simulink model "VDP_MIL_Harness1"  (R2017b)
settings: Solver=FixedStepDiscrete  StartTime=0.0  StopTime=50  FixedStep=0.01  RelTol=1e-3  EnableMultiTasking=on
undefined symbols (not defined in the file): sigbuilder_block

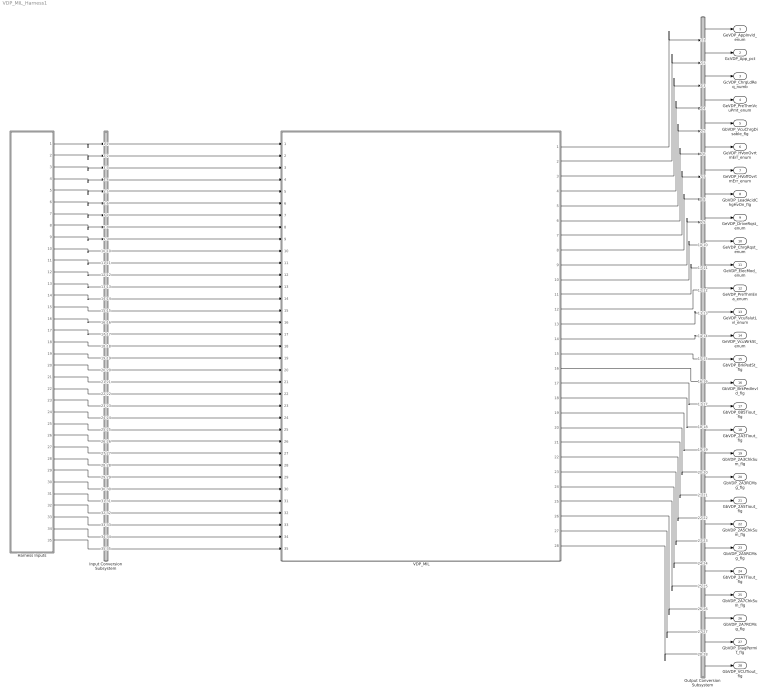
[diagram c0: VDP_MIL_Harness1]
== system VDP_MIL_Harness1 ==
  Harness Inputs : Subsystem  Tag=STV Subsys  LoadFcn=sigbuilder_block('load');  StartFcn=sigbuilder_block('start');  StopFcn=sigbuilder_block('stop');  ClipboardFcn=sigbuilder_block('clipboard');  mask(Sigbuilder block){tuvar=[0:10]}
      mask init:
      | if ~strcmp(get_param(bdroot(gcb),'SimulationStatus'),'stopped'),tuvar = sigbuilder_block('maskInit'); end
  Input Conversion Subsystem : Subsystem  Tag=__SLT_ICS__  Description=Signal spec. and routing
  Output Conversion Subsystem : Subsystem  Tag=__SLT_OCS__  Description=Signal spec. and routing
  VDP_MIL : ModelReference  ModelNameDialog=VDP_MIL  SimulationMode=Normal  ModelReferenceVersion='M107C106'
  GeVDP_AppInvld_enum : Outport  OutDataTypeStr=uint8  PortDimensions=[1]
  GcVDP_App_pct : Outport  Port=2  OutDataTypeStr=single  PortDimensions=[1]
  GcVDP_ChrgLdReq_numb : Outport  Port=3  OutDataTypeStr=single  PortDimensions=[1]
  GeVDP_PreThmVcuPmt_enum : Outport  Port=4  OutDataTypeStr=uint8  PortDimensions=[1]
  GbVDP_VcuChrgDisable_flg : Outport  Port=5  OutDataTypeStr=boolean  PortDimensions=[1]
  GeVDP_HVonOvrtmErr_enum : Outport  Port=6  OutDataTypeStr=uint8  PortDimensions=[1]
  GeVDP_HVoffOvrtmErr_enum : Outport  Port=7  OutDataTypeStr=uint8  PortDimensions=[1]
  GbVDP_LeadAcidChgHvOn_flg : Outport  Port=8  OutDataTypeStr=boolean  PortDimensions=[1]
  GeVDP_DriveRqst_enum : Outport  Port=9  OutDataTypeStr=uint8  PortDimensions=[1]
  GeVDP_ChrgRqst_enum : Outport  Port=10  OutDataTypeStr=uint8  PortDimensions=[1]
  GeVDP_ElecMod_enum : Outport  Port=11  OutDataTypeStr=uint8  PortDimensions=[1]
  GeVDP_PreThmEna_enum : Outport  Port=12  OutDataTypeStr=uint8  PortDimensions=[1]
  GeVDP_VcuFalutLvl_enum : Outport  Port=13  OutDataTypeStr=uint8  PortDimensions=[1]
  GeVDP_VcuWrkSt_enum : Outport  Port=14  OutDataTypeStr=uint8  PortDimensions=[1]
  GbVDP_BrkPedSt_flg : Outport  Port=15  OutDataTypeStr=boolean  PortDimensions=[1]
  GbVDP_BrkPedInvld_flg : Outport  Port=16  OutDataTypeStr=boolean  PortDimensions=[1]
  GbVDP_0B5Tiout_flg : Outport  Port=17  OutDataTypeStr=boolean  PortDimensions=[1]
  GbVDP_2A3Tiout_flg : Outport  Port=18  OutDataTypeStr=boolean  PortDimensions=[1]
  GbVDP_2A3ChkSum_flg : Outport  Port=19  OutDataTypeStr=boolean  PortDimensions=[1]
  GbVDP_2A3RCMsg_flg : Outport  Port=20  OutDataTypeStr=boolean  PortDimensions=[1]
  GbVDP_2A5Tiout_flg : Outport  Port=21  OutDataTypeStr=boolean  PortDimensions=[1]
  GbVDP_2A5ChkSum_flg : Outport  Port=22  OutDataTypeStr=boolean  PortDimensions=[1]
  GbVDP_2A5RCMsg_flg : Outport  Port=23  OutDataTypeStr=boolean  PortDimensions=[1]
  GbVDP_2A7Tiout_flg : Outport  Port=24  OutDataTypeStr=boolean  PortDimensions=[1]
  GbVDP_2A7ChkSum_flg : Outport  Port=25  OutDataTypeStr=boolean  PortDimensions=[1]
  GbVDP_2A7RCMsg_flg : Outport  Port=26  OutDataTypeStr=boolean  PortDimensions=[1]
  GbVDP_DiagPermit_flg : Outport  Port=27  OutDataTypeStr=boolean  PortDimensions=[1]
  GbVDP_VCUTiout_flg : Outport  Port=28  OutDataTypeStr=boolean  PortDimensions=[1]
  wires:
  Harness Inputs/1(GeISP_AppInvld_enum) -> Input Conversion Subsystem/1(Inport_1)
  Harness Inputs/2(GcISP_App_pct) -> Input Conversion Subsystem/2(Inport_2)
  Harness Inputs/3(GbISP_0B5Tiout_flg) -> Input Conversion Subsystem/3(Inport_3)
  Harness Inputs/4(GcISP_ChrgLdReq_numb) -> Input Conversion Subsystem/4(Inport_4)
  Harness Inputs/5(GeISP_VcuPwrReqBatA_enum) -> Input Conversion Subsystem/5(Inport_5)
  Harness Inputs/6(GeISP_PreThmVcuPmt_enum) -> Input Conversion Subsystem/6(Inport_6)
  Harness Inputs/7(GbISP_VcuChrgDisable_flg) -> Input Conversion Subsystem/7(Inport_7)
  Harness Inputs/8(GeISP_HVonOvrtmErr_enum) -> Input Conversion Subsystem/8(Inport_8)
  Harness Inputs/9(GeISP_HVoffOvrtmErr_enum) -> Input Conversion Subsystem/9(Inport_9)
  Harness Inputs/10(GbISP_LeadAcidChgHvOn_flg) -> Input Conversion Subsystem/10(Inport_10)
  Harness Inputs/11(GbISP_2A3Tiout_flg) -> Input Conversion Subsystem/11(Inport_11)
  Harness Inputs/12(GeISP_ElecMod_enum) -> Input Conversion Subsystem/12(Inport_12)
  Harness Inputs/13(GeISP_PreThmEna_enum) -> Input Conversion Subsystem/13(Inport_13)
  Harness Inputs/14(GbISP_2A5Tiout_flg) -> Input Conversion Subsystem/14(Inport_14)
  Harness Inputs/15(GeISP_VcuFalutLvl_enum) -> Input Conversion Subsystem/15(Inport_15)
  Harness Inputs/16(GeISP_VcuWrkSt_enum) -> Input Conversion Subsystem/16(Inport_16)
  Harness Inputs/17(GbISP_BrkPedSt_flg) -> Input Conversion Subsystem/17(Inport_17)
  Harness Inputs/18(GbISP_BrkPedInvld_flg) -> Input Conversion Subsystem/18(Inport_18)
  Harness Inputs/19(GbISP_2A7Tiout_flg) -> Input Conversion Subsystem/19(Inport_19)
  Harness Inputs/20(GbISP_PtCANBusoff_flg) -> Input Conversion Subsystem/20(Inport_20)
  Harness Inputs/21(GcLDP_Kl30Volt_mV) -> Input Conversion Subsystem/21(Inport_21)
  Harness Inputs/22(GcADP_YearSet_Yr) -> Input Conversion Subsystem/22(Inport_22)
  Harness Inputs/23(GbADP_OTAmodeONReq_flg) -> Input Conversion Subsystem/23(Inport_23)
  Harness Inputs/24(GbISP_DiagModeONReq_flg) -> Input Conversion Subsystem/24(Inport_24)
  Harness Inputs/25(GbISP_ChkSumMsg2A3Err_flg) -> Input Conversion Subsystem/25(Inport_25)
  Harness Inputs/26(GbISP_RcMsg2A3Err_flg) -> Input Conversion Subsystem/26(Inport_26)
  Harness Inputs/27(GbISP_ChkSumMsg2A5Err_flg) -> Input Conversion Subsystem/27(Inport_27)
  Harness Inputs/28(GbISP_RcMsg2A5Err_flg) -> Input Conversion Subsystem/28(Inport_28)
  Harness Inputs/29(GbISP_ChkSumMsg2A7Err_flg) -> Input Conversion Subsystem/29(Inport_29)
  Harness Inputs/30(GbISP_RcMsg2A7Err_flg) -> Input Conversion Subsystem/30(Inport_30)
  Harness Inputs/31(GbISP_Kl15WkUp_flg) -> Input Conversion Subsystem/31(Inport_31)
  Harness Inputs/32(GbWSM_ACWkUpPrs_flg) -> Input Conversion Subsystem/32(Inport_32)
  Harness Inputs/33(GbWSM_DCWkUpPrs_flg) -> Input Conversion Subsystem/33(Inport_33)
  Harness Inputs/34(GbWSM_EDCWkUpPrs_flg) -> Input Conversion Subsystem/34(Inport_34)
  Harness Inputs/35(GbWSM_CANWkUpPrs_flg) -> Input Conversion Subsystem/35(Inport_35)
  Output Conversion Subsystem/1(Outport_1) -> GeVDP_AppInvld_enum/1
  Output Conversion Subsystem/2(Outport_2) -> GcVDP_App_pct/1
  Output Conversion Subsystem/3(Outport_3) -> GcVDP_ChrgLdReq_numb/1
  Output Conversion Subsystem/4(Outport_4) -> GeVDP_PreThmVcuPmt_enum/1
  Output Conversion Subsystem/5(Outport_5) -> GbVDP_VcuChrgDisable_flg/1
  Output Conversion Subsystem/6(Outport_6) -> GeVDP_HVonOvrtmErr_enum/1
  Output Conversion Subsystem/7(Outport_7) -> GeVDP_HVoffOvrtmErr_enum/1
  Output Conversion Subsystem/8(Outport_8) -> GbVDP_LeadAcidChgHvOn_flg/1
  Output Conversion Subsystem/9(Outport_9) -> GeVDP_DriveRqst_enum/1
  Output Conversion Subsystem/10(Outport_10) -> GeVDP_ChrgRqst_enum/1
  Output Conversion Subsystem/11(Outport_11) -> GeVDP_ElecMod_enum/1
  Output Conversion Subsystem/12(Outport_12) -> GeVDP_PreThmEna_enum/1
  Output Conversion Subsystem/13(Outport_13) -> GeVDP_VcuFalutLvl_enum/1
  Output Conversion Subsystem/14(Outport_14) -> GeVDP_VcuWrkSt_enum/1
  Output Conversion Subsystem/15(Outport_15) -> GbVDP_BrkPedSt_flg/1
  Output Conversion Subsystem/16(Outport_16) -> GbVDP_BrkPedInvld_flg/1
  Output Conversion Subsystem/17(Outport_17) -> GbVDP_0B5Tiout_flg/1
  Output Conversion Subsystem/18(Outport_18) -> GbVDP_2A3Tiout_flg/1
  Output Conversion Subsystem/19(Outport_19) -> GbVDP_2A3ChkSum_flg/1
  Output Conversion Subsystem/20(Outport_20) -> GbVDP_2A3RCMsg_flg/1
  Output Conversion Subsystem/21(Outport_21) -> GbVDP_2A5Tiout_flg/1
  Output Conversion Subsystem/22(Outport_22) -> GbVDP_2A5ChkSum_flg/1
  Output Conversion Subsystem/23(Outport_23) -> GbVDP_2A5RCMsg_flg/1
  Output Conversion Subsystem/24(Outport_24) -> GbVDP_2A7Tiout_flg/1
  Output Conversion Subsystem/25(Outport_25) -> GbVDP_2A7ChkSum_flg/1
  Output Conversion Subsystem/26(Outport_26) -> GbVDP_2A7RCMsg_flg/1
  Output Conversion Subsystem/27(Outport_27) -> GbVDP_DiagPermit_flg/1
  Output Conversion Subsystem/28(Outport_28) -> GbVDP_VCUTiout_flg/1
  Input Conversion Subsystem/1(Outport_1) -> VDP_MIL/1
  Input Conversion Subsystem/2(Outport_2) -> VDP_MIL/2
  Input Conversion Subsystem/3(Outport_3) -> VDP_MIL/3
  Input Conversion Subsystem/4(Outport_4) -> VDP_MIL/4
  Input Conversion Subsystem/5(Outport_5) -> VDP_MIL/5
  Input Conversion Subsystem/6(Outport_6) -> VDP_MIL/6
  Input Conversion Subsystem/7(Outport_7) -> VDP_MIL/7
  Input Conversion Subsystem/8(Outport_8) -> VDP_MIL/8
  Input Conversion Subsystem/9(Outport_9) -> VDP_MIL/9
  Input Conversion Subsystem/10(Outport_10) -> VDP_MIL/10
  Input Conversion Subsystem/11(Outport_11) -> VDP_MIL/11
  Input Conversion Subsystem/12(Outport_12) -> VDP_MIL/12
  Input Conversion Subsystem/13(Outport_13) -> VDP_MIL/13
  Input Conversion Subsystem/14(Outport_14) -> VDP_MIL/14
  Input Conversion Subsystem/15(Outport_15) -> VDP_MIL/15
  Input Conversion Subsystem/16(Outport_16) -> VDP_MIL/16
  Input Conversion Subsystem/17(Outport_17) -> VDP_MIL/17
  Input Conversion Subsystem/18(Outport_18) -> VDP_MIL/18
  Input Conversion Subsystem/19(Outport_19) -> VDP_MIL/19
  Input Conversion Subsystem/20(Outport_20) -> VDP_MIL/20
  Input Conversion Subsystem/21(Outport_21) -> VDP_MIL/21
  Input Conversion Subsystem/22(Outport_22) -> VDP_MIL/22
  Input Conversion Subsystem/23(Outport_23) -> VDP_MIL/23
  Input Conversion Subsystem/24(Outport_24) -> VDP_MIL/24
  Input Conversion Subsystem/25(Outport_25) -> VDP_MIL/25
  Input Conversion Subsystem/26(Outport_26) -> VDP_MIL/26
  Input Conversion Subsystem/27(Outport_27) -> VDP_MIL/27
  Input Conversion Subsystem/28(Outport_28) -> VDP_MIL/28
  Input Conversion Subsystem/29(Outport_29) -> VDP_MIL/29
  Input Conversion Subsystem/30(Outport_30) -> VDP_MIL/30
  Input Conversion Subsystem/31(Outport_31) -> VDP_MIL/31
  Input Conversion Subsystem/32(Outport_32) -> VDP_MIL/32
  Input Conversion Subsystem/33(Outport_33) -> VDP_MIL/33
  Input Conversion Subsystem/34(Outport_34) -> VDP_MIL/34
  Input Conversion Subsystem/35(Outport_35) -> VDP_MIL/35
  VDP_MIL/1 -> Output Conversion Subsystem/1(Inport_1)
  VDP_MIL/2 -> Output Conversion Subsystem/2(Inport_2)
  VDP_MIL/3 -> Output Conversion Subsystem/3(Inport_3)
  VDP_MIL/4 -> Output Conversion Subsystem/4(Inport_4)
  VDP_MIL/5 -> Output Conversion Subsystem/5(Inport_5)
  VDP_MIL/6 -> Output Conversion Subsystem/6(Inport_6)
  VDP_MIL/7 -> Output Conversion Subsystem/7(Inport_7)
  VDP_MIL/8 -> Output Conversion Subsystem/8(Inport_8)
  VDP_MIL/9 -> Output Conversion Subsystem/9(Inport_9)
  VDP_MIL/10 -> Output Conversion Subsystem/10(Inport_10)
  VDP_MIL/11 -> Output Conversion Subsystem/11(Inport_11)
  VDP_MIL/12 -> Output Conversion Subsystem/12(Inport_12)
  VDP_MIL/13 -> Output Conversion Subsystem/13(Inport_13)
  VDP_MIL/14 -> Output Conversion Subsystem/14(Inport_14)
  VDP_MIL/15 -> Output Conversion Subsystem/15(Inport_15)
  VDP_MIL/16 -> Output Conversion Subsystem/16(Inport_16)
  VDP_MIL/17 -> Output Conversion Subsystem/17(Inport_17)
  VDP_MIL/18 -> Output Conversion Subsystem/18(Inport_18)
  VDP_MIL/19 -> Output Conversion Subsystem/19(Inport_19)
  VDP_MIL/20 -> Output Conversion Subsystem/20(Inport_20)
  VDP_MIL/21 -> Output Conversion Subsystem/21(Inport_21)
  VDP_MIL/22 -> Output Conversion Subsystem/22(Inport_22)
  VDP_MIL/23 -> Output Conversion Subsystem/23(Inport_23)
  VDP_MIL/24 -> Output Conversion Subsystem/24(Inport_24)
  VDP_MIL/25 -> Output Conversion Subsystem/25(Inport_25)
  VDP_MIL/26 -> Output Conversion Subsystem/26(Inport_26)
  VDP_MIL/27 -> Output Conversion Subsystem/27(Inport_27)
  VDP_MIL/28 -> Output Conversion Subsystem/28(Inport_28)

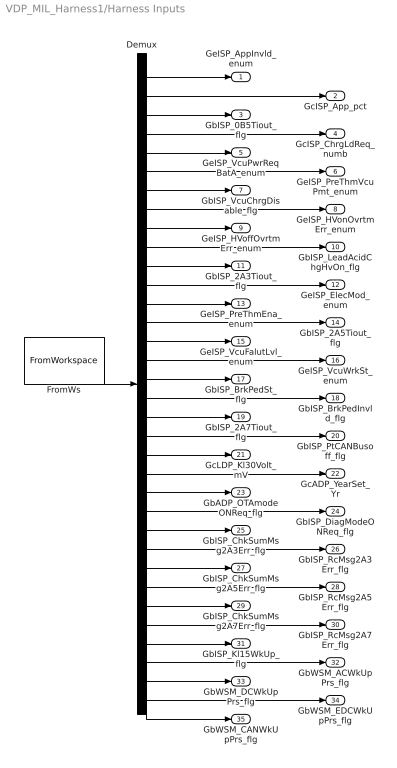
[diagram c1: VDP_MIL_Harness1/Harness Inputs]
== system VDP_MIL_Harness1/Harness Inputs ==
  Demux : Demux  Tag=STV Demux  Outputs=35
  FromWs : FromWorkspace  Tag=STV FromWs  VariableName=tuvar  SampleTime=0
  GeISP_AppInvld_enum : Outport  Tag=STV Outport
  GcISP_App_pct : Outport  Tag=STV Outport  Port=2
  GbISP_0B5Tiout_flg : Outport  Tag=STV Outport  Port=3
  GcISP_ChrgLdReq_numb : Outport  Tag=STV Outport  Port=4
  GeISP_VcuPwrReqBatA_enum : Outport  Tag=STV Outport  Port=5
  GeISP_PreThmVcuPmt_enum : Outport  Tag=STV Outport  Port=6
  GbISP_VcuChrgDisable_flg : Outport  Tag=STV Outport  Port=7
  GeISP_HVonOvrtmErr_enum : Outport  Tag=STV Outport  Port=8
  GeISP_HVoffOvrtmErr_enum : Outport  Tag=STV Outport  Port=9
  GbISP_LeadAcidChgHvOn_flg : Outport  Tag=STV Outport  Port=10
  GbISP_2A3Tiout_flg : Outport  Tag=STV Outport  Port=11
  GeISP_ElecMod_enum : Outport  Tag=STV Outport  Port=12
  GeISP_PreThmEna_enum : Outport  Tag=STV Outport  Port=13
  GbISP_2A5Tiout_flg : Outport  Tag=STV Outport  Port=14
  GeISP_VcuFalutLvl_enum : Outport  Tag=STV Outport  Port=15
  GeISP_VcuWrkSt_enum : Outport  Tag=STV Outport  Port=16
  GbISP_BrkPedSt_flg : Outport  Tag=STV Outport  Port=17
  GbISP_BrkPedInvld_flg : Outport  Tag=STV Outport  Port=18
  GbISP_2A7Tiout_flg : Outport  Tag=STV Outport  Port=19
  GbISP_PtCANBusoff_flg : Outport  Tag=STV Outport  Port=20
  GcLDP_Kl30Volt_mV : Outport  Tag=STV Outport  Port=21
  GcADP_YearSet_Yr : Outport  Tag=STV Outport  Port=22
  GbADP_OTAmodeONReq_flg : Outport  Tag=STV Outport  Port=23
  GbISP_DiagModeONReq_flg : Outport  Tag=STV Outport  Port=24
  GbISP_ChkSumMsg2A3Err_flg : Outport  Tag=STV Outport  Port=25
  GbISP_RcMsg2A3Err_flg : Outport  Tag=STV Outport  Port=26
  GbISP_ChkSumMsg2A5Err_flg : Outport  Tag=STV Outport  Port=27
  GbISP_RcMsg2A5Err_flg : Outport  Tag=STV Outport  Port=28
  GbISP_ChkSumMsg2A7Err_flg : Outport  Tag=STV Outport  Port=29
  GbISP_RcMsg2A7Err_flg : Outport  Tag=STV Outport  Port=30
  GbISP_Kl15WkUp_flg : Outport  Tag=STV Outport  Port=31
  GbWSM_ACWkUpPrs_flg : Outport  Tag=STV Outport  Port=32
  GbWSM_DCWkUpPrs_flg : Outport  Tag=STV Outport  Port=33
  GbWSM_EDCWkUpPrs_flg : Outport  Tag=STV Outport  Port=34
  GbWSM_CANWkUpPrs_flg : Outport  Tag=STV Outport  Port=35
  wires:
  FromWs/1 -> Demux/1
  Demux/1 -> GeISP_AppInvld_enum/1
  Demux/2 -> GcISP_App_pct/1
  Demux/3 -> GbISP_0B5Tiout_flg/1
  Demux/4 -> GcISP_ChrgLdReq_numb/1
  Demux/5 -> GeISP_VcuPwrReqBatA_enum/1
  Demux/6 -> GeISP_PreThmVcuPmt_enum/1
  Demux/7 -> GbISP_VcuChrgDisable_flg/1
  Demux/8 -> GeISP_HVonOvrtmErr_enum/1
  Demux/9 -> GeISP_HVoffOvrtmErr_enum/1
  Demux/10 -> GbISP_LeadAcidChgHvOn_flg/1
  Demux/11 -> GbISP_2A3Tiout_flg/1
  Demux/12 -> GeISP_ElecMod_enum/1
  Demux/13 -> GeISP_PreThmEna_enum/1
  Demux/14 -> GbISP_2A5Tiout_flg/1
  Demux/15 -> GeISP_VcuFalutLvl_enum/1
  Demux/16 -> GeISP_VcuWrkSt_enum/1
  Demux/17 -> GbISP_BrkPedSt_flg/1
  Demux/18 -> GbISP_BrkPedInvld_flg/1
  Demux/19 -> GbISP_2A7Tiout_flg/1
  Demux/20 -> GbISP_PtCANBusoff_flg/1
  Demux/21 -> GcLDP_Kl30Volt_mV/1
  Demux/22 -> GcADP_YearSet_Yr/1
  Demux/23 -> GbADP_OTAmodeONReq_flg/1
  Demux/24 -> GbISP_DiagModeONReq_flg/1
  Demux/25 -> GbISP_ChkSumMsg2A3Err_flg/1
  Demux/26 -> GbISP_RcMsg2A3Err_flg/1
  Demux/27 -> GbISP_ChkSumMsg2A5Err_flg/1
  Demux/28 -> GbISP_RcMsg2A5Err_flg/1
  Demux/29 -> GbISP_ChkSumMsg2A7Err_flg/1
  Demux/30 -> GbISP_RcMsg2A7Err_flg/1
  Demux/31 -> GbISP_Kl15WkUp_flg/1
  Demux/32 -> GbWSM_ACWkUpPrs_flg/1
  Demux/33 -> GbWSM_DCWkUpPrs_flg/1
  Demux/34 -> GbWSM_EDCWkUpPrs_flg/1
  Demux/35 -> GbWSM_CANWkUpPrs_flg/1

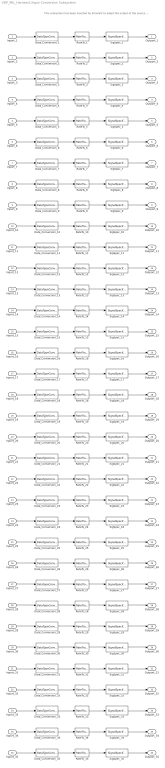
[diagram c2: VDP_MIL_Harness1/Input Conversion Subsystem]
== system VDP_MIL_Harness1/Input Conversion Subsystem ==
  note: This subsystem has been inserted by Simulink to adapt the output of the source blocks to the interface required by the harnessed component. Modifying the contents of this subsystem may result in compilation and simulation failure.
  Inport_1 : Inport
  Inport_2 : Inport  Port=2
  Inport_3 : Inport  Port=3
  Inport_4 : Inport  Port=4
  Inport_5 : Inport  Port=5
  Inport_6 : Inport  Port=6
  Inport_7 : Inport  Port=7
  Inport_8 : Inport  Port=8
  Inport_9 : Inport  Port=9
  Inport_10 : Inport  Port=10
  Inport_11 : Inport  Port=11
  Inport_12 : Inport  Port=12
  Inport_13 : Inport  Port=13
  Inport_14 : Inport  Port=14
  Inport_15 : Inport  Port=15
  Inport_16 : Inport  Port=16
  Inport_17 : Inport  Port=17
  Inport_18 : Inport  Port=18
  Inport_19 : Inport  Port=19
  Inport_20 : Inport  Port=20
  Inport_21 : Inport  Port=21
  Inport_22 : Inport  Port=22
  Inport_23 : Inport  Port=23
  Inport_24 : Inport  Port=24
  Inport_25 : Inport  Port=25
  Inport_26 : Inport  Port=26
  Inport_27 : Inport  Port=27
  Inport_28 : Inport  Port=28
  Inport_29 : Inport  Port=29
  Inport_30 : Inport  Port=30
  Inport_31 : Inport  Port=31
  Inport_32 : Inport  Port=32
  Inport_33 : Inport  Port=33
  Inport_34 : Inport  Port=34
  Inport_35 : Inport  Port=35
  Data_Conversion_{1,5..6,8..9,12..13,15..16} (9 alike) : DataTypeConversion  OutDataTypeStr=uint8
  Data_Conversion_{3,7,10..11,14,17..20,23..35} (22 alike) : DataTypeConversion  OutDataTypeStr=boolean
  Data_Conversion_2 : DataTypeConversion  OutDataTypeStr=fixdt('ufix8_Sp4')
  Data_Conversion_21 : DataTypeConversion  OutDataTypeStr=uint16
  Data_Conversion_22 : DataTypeConversion  OutDataTypeStr=uint16
  Data_Conversion_4 : DataTypeConversion  OutDataTypeStr=fixdt('ufix8_Sp1')
  RateTs_{1..35} (35 alike) : RateTransition  OutPortSampleTime=0.01
  SigSpec_{1,5..6,8..9,12..13,15..16} (9 alike) : SignalSpecification  OutDataTypeStr=uint8  Unit=enum  Dimensions=[1]  SampleTime=0.01
  SigSpec_{3,7,10..11,14,17..20,24..31} (17 alike) : SignalSpecification  OutDataTypeStr=boolean  Unit=flag  Dimensions=[1]  SampleTime=0.01
  SigSpec_2 : SignalSpecification  OutDataTypeStr=fixdt('ufix8_Sp4')  Unit=%  Dimensions=[1]  SampleTime=0.01
  SigSpec_21 : SignalSpecification  OutDataTypeStr=uint16  Unit=mv  Dimensions=[1]  SampleTime=0.01
  SigSpec_22 : SignalSpecification  OutDataTypeStr=uint16  Unit=Yr  Dimensions=[1]  SampleTime=0.01
  SigSpec_{23,32..35} (5 alike) : SignalSpecification  OutDataTypeStr=boolean  Unit=flg  Dimensions=[1]  SampleTime=0.01
  SigSpec_4 : SignalSpecification  OutDataTypeStr=fixdt('ufix8_Sp1')  Unit=numb  Dimensions=[1]  SampleTime=0.01
  Outport_1 : Outport
  Outport_2 : Outport  Port=2
  Outport_3 : Outport  Port=3
  Outport_4 : Outport  Port=4
  Outport_5 : Outport  Port=5
  Outport_6 : Outport  Port=6
  Outport_7 : Outport  Port=7
  Outport_8 : Outport  Port=8
  Outport_9 : Outport  Port=9
  Outport_10 : Outport  Port=10
  Outport_11 : Outport  Port=11
  Outport_12 : Outport  Port=12
  Outport_13 : Outport  Port=13
  Outport_14 : Outport  Port=14
  Outport_15 : Outport  Port=15
  Outport_16 : Outport  Port=16
  Outport_17 : Outport  Port=17
  Outport_18 : Outport  Port=18
  Outport_19 : Outport  Port=19
  Outport_20 : Outport  Port=20
  Outport_21 : Outport  Port=21
  Outport_22 : Outport  Port=22
  Outport_23 : Outport  Port=23
  Outport_24 : Outport  Port=24
  Outport_25 : Outport  Port=25
  Outport_26 : Outport  Port=26
  Outport_27 : Outport  Port=27
  Outport_28 : Outport  Port=28
  Outport_29 : Outport  Port=29
  Outport_30 : Outport  Port=30
  Outport_31 : Outport  Port=31
  Outport_32 : Outport  Port=32
  Outport_33 : Outport  Port=33
  Outport_34 : Outport  Port=34
  Outport_35 : Outport  Port=35
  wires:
  SigSpec_1/1 -> Outport_1/1
  RateTs_1/1 -> SigSpec_1/1
  Data_Conversion_1/1 -> RateTs_1/1
  Inport_1/1 -> Data_Conversion_1/1
  SigSpec_2/1 -> Outport_2/1
  RateTs_2/1 -> SigSpec_2/1
  Data_Conversion_2/1 -> RateTs_2/1
  Inport_2/1 -> Data_Conversion_2/1
  SigSpec_3/1 -> Outport_3/1
  RateTs_3/1 -> SigSpec_3/1
  Data_Conversion_3/1 -> RateTs_3/1
  Inport_3/1 -> Data_Conversion_3/1
  SigSpec_4/1 -> Outport_4/1
  RateTs_4/1 -> SigSpec_4/1
  Data_Conversion_4/1 -> RateTs_4/1
  Inport_4/1 -> Data_Conversion_4/1
  SigSpec_5/1 -> Outport_5/1
  RateTs_5/1 -> SigSpec_5/1
  Data_Conversion_5/1 -> RateTs_5/1
  Inport_5/1 -> Data_Conversion_5/1
  SigSpec_6/1 -> Outport_6/1
  RateTs_6/1 -> SigSpec_6/1
  Data_Conversion_6/1 -> RateTs_6/1
  Inport_6/1 -> Data_Conversion_6/1
  SigSpec_7/1 -> Outport_7/1
  RateTs_7/1 -> SigSpec_7/1
  Data_Conversion_7/1 -> RateTs_7/1
  Inport_7/1 -> Data_Conversion_7/1
  SigSpec_8/1 -> Outport_8/1
  RateTs_8/1 -> SigSpec_8/1
  Data_Conversion_8/1 -> RateTs_8/1
  Inport_8/1 -> Data_Conversion_8/1
  SigSpec_9/1 -> Outport_9/1
  RateTs_9/1 -> SigSpec_9/1
  Data_Conversion_9/1 -> RateTs_9/1
  Inport_9/1 -> Data_Conversion_9/1
  SigSpec_10/1 -> Outport_10/1
  RateTs_10/1 -> SigSpec_10/1
  Data_Conversion_10/1 -> RateTs_10/1
  Inport_10/1 -> Data_Conversion_10/1
  SigSpec_11/1 -> Outport_11/1
  RateTs_11/1 -> SigSpec_11/1
  Data_Conversion_11/1 -> RateTs_11/1
  Inport_11/1 -> Data_Conversion_11/1
  SigSpec_12/1 -> Outport_12/1
  RateTs_12/1 -> SigSpec_12/1
  Data_Conversion_12/1 -> RateTs_12/1
  Inport_12/1 -> Data_Conversion_12/1
  SigSpec_13/1 -> Outport_13/1
  RateTs_13/1 -> SigSpec_13/1
  Data_Conversion_13/1 -> RateTs_13/1
  Inport_13/1 -> Data_Conversion_13/1
  SigSpec_14/1 -> Outport_14/1
  RateTs_14/1 -> SigSpec_14/1
  Data_Conversion_14/1 -> RateTs_14/1
  Inport_14/1 -> Data_Conversion_14/1
  SigSpec_15/1 -> Outport_15/1
  RateTs_15/1 -> SigSpec_15/1
  Data_Conversion_15/1 -> RateTs_15/1
  Inport_15/1 -> Data_Conversion_15/1
  SigSpec_16/1 -> Outport_16/1
  RateTs_16/1 -> SigSpec_16/1
  Data_Conversion_16/1 -> RateTs_16/1
  Inport_16/1 -> Data_Conversion_16/1
  SigSpec_17/1 -> Outport_17/1
  RateTs_17/1 -> SigSpec_17/1
  Data_Conversion_17/1 -> RateTs_17/1
  Inport_17/1 -> Data_Conversion_17/1
  SigSpec_18/1 -> Outport_18/1
  RateTs_18/1 -> SigSpec_18/1
  Data_Conversion_18/1 -> RateTs_18/1
  Inport_18/1 -> Data_Conversion_18/1
  SigSpec_19/1 -> Outport_19/1
  RateTs_19/1 -> SigSpec_19/1
  Data_Conversion_19/1 -> RateTs_19/1
  Inport_19/1 -> Data_Conversion_19/1
  SigSpec_20/1 -> Outport_20/1
  RateTs_20/1 -> SigSpec_20/1
  Data_Conversion_20/1 -> RateTs_20/1
  Inport_20/1 -> Data_Conversion_20/1
  SigSpec_21/1 -> Outport_21/1
  RateTs_21/1 -> SigSpec_21/1
  Data_Conversion_21/1 -> RateTs_21/1
  Inport_21/1 -> Data_Conversion_21/1
  SigSpec_22/1 -> Outport_22/1
  RateTs_22/1 -> SigSpec_22/1
  Data_Conversion_22/1 -> RateTs_22/1
  Inport_22/1 -> Data_Conversion_22/1
  SigSpec_23/1 -> Outport_23/1
  RateTs_23/1 -> SigSpec_23/1
  Data_Conversion_23/1 -> RateTs_23/1
  Inport_23/1 -> Data_Conversion_23/1
  SigSpec_24/1 -> Outport_24/1
  RateTs_24/1 -> SigSpec_24/1
  Data_Conversion_24/1 -> RateTs_24/1
  Inport_24/1 -> Data_Conversion_24/1
  SigSpec_25/1 -> Outport_25/1
  RateTs_25/1 -> SigSpec_25/1
  Data_Conversion_25/1 -> RateTs_25/1
  Inport_25/1 -> Data_Conversion_25/1
  SigSpec_26/1 -> Outport_26/1
  RateTs_26/1 -> SigSpec_26/1
  Data_Conversion_26/1 -> RateTs_26/1
  Inport_26/1 -> Data_Conversion_26/1
  SigSpec_27/1 -> Outport_27/1
  RateTs_27/1 -> SigSpec_27/1
  Data_Conversion_27/1 -> RateTs_27/1
  Inport_27/1 -> Data_Conversion_27/1
  SigSpec_28/1 -> Outport_28/1
  RateTs_28/1 -> SigSpec_28/1
  Data_Conversion_28/1 -> RateTs_28/1
  Inport_28/1 -> Data_Conversion_28/1
  SigSpec_29/1 -> Outport_29/1
  RateTs_29/1 -> SigSpec_29/1
  Data_Conversion_29/1 -> RateTs_29/1
  Inport_29/1 -> Data_Conversion_29/1
  SigSpec_30/1 -> Outport_30/1
  RateTs_30/1 -> SigSpec_30/1
  Data_Conversion_30/1 -> RateTs_30/1
  Inport_30/1 -> Data_Conversion_30/1
  SigSpec_31/1 -> Outport_31/1
  RateTs_31/1 -> SigSpec_31/1
  Data_Conversion_31/1 -> RateTs_31/1
  Inport_31/1 -> Data_Conversion_31/1
  SigSpec_32/1 -> Outport_32/1
  RateTs_32/1 -> SigSpec_32/1
  Data_Conversion_32/1 -> RateTs_32/1
  Inport_32/1 -> Data_Conversion_32/1
  SigSpec_33/1 -> Outport_33/1
  RateTs_33/1 -> SigSpec_33/1
  Data_Conversion_33/1 -> RateTs_33/1
  Inport_33/1 -> Data_Conversion_33/1
  SigSpec_34/1 -> Outport_34/1
  RateTs_34/1 -> SigSpec_34/1
  Data_Conversion_34/1 -> RateTs_34/1
  Inport_34/1 -> Data_Conversion_34/1
  SigSpec_35/1 -> Outport_35/1
  RateTs_35/1 -> SigSpec_35/1
  Data_Conversion_35/1 -> RateTs_35/1
  Inport_35/1 -> Data_Conversion_35/1

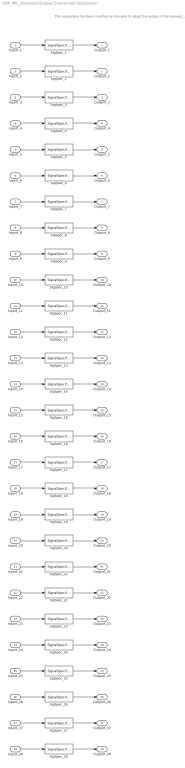
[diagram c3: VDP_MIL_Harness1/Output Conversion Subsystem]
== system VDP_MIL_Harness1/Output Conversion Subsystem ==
  note: This subsystem has been inserted by Simulink to adapt the output of the harnessed component to the interface required by the sink blocks. Modifying the contents of this subsystem may result in compilation and simulation failure.
  Inport_1 : Inport
  Inport_2 : Inport  Port=2
  Inport_3 : Inport  Port=3
  Inport_4 : Inport  Port=4
  Inport_5 : Inport  Port=5
  Inport_6 : Inport  Port=6
  Inport_7 : Inport  Port=7
  Inport_8 : Inport  Port=8
  Inport_9 : Inport  Port=9
  Inport_10 : Inport  Port=10
  Inport_11 : Inport  Port=11
  Inport_12 : Inport  Port=12
  Inport_13 : Inport  Port=13
  Inport_14 : Inport  Port=14
  Inport_15 : Inport  Port=15
  Inport_16 : Inport  Port=16
  Inport_17 : Inport  Port=17
  Inport_18 : Inport  Port=18
  Inport_19 : Inport  Port=19
  Inport_20 : Inport  Port=20
  Inport_21 : Inport  Port=21
  Inport_22 : Inport  Port=22
  Inport_23 : Inport  Port=23
  Inport_24 : Inport  Port=24
  Inport_25 : Inport  Port=25
  Inport_26 : Inport  Port=26
  Inport_27 : Inport  Port=27
  Inport_28 : Inport  Port=28
  SigSpec_{1,4,6..7,9..14} (10 alike) : SignalSpecification  OutDataTypeStr=uint8  Unit=enum  Dimensions=[1]  SampleTime=0.01
  SigSpec_{5,8,15..28} (16 alike) : SignalSpecification  OutDataTypeStr=boolean  Unit=flg  Dimensions=[1]  SampleTime=0.01
  SigSpec_2 : SignalSpecification  OutDataTypeStr=single  Unit=%  Dimensions=[1]  SampleTime=0.01
  SigSpec_3 : SignalSpecification  OutDataTypeStr=single  Unit=kW  Dimensions=[1]  SampleTime=0.01
  Outport_1 : Outport
  Outport_2 : Outport  Port=2
  Outport_3 : Outport  Port=3
  Outport_4 : Outport  Port=4
  Outport_5 : Outport  Port=5
  Outport_6 : Outport  Port=6
  Outport_7 : Outport  Port=7
  Outport_8 : Outport  Port=8
  Outport_9 : Outport  Port=9
  Outport_10 : Outport  Port=10
  Outport_11 : Outport  Port=11
  Outport_12 : Outport  Port=12
  Outport_13 : Outport  Port=13
  Outport_14 : Outport  Port=14
  Outport_15 : Outport  Port=15
  Outport_16 : Outport  Port=16
  Outport_17 : Outport  Port=17
  Outport_18 : Outport  Port=18
  Outport_19 : Outport  Port=19
  Outport_20 : Outport  Port=20
  Outport_21 : Outport  Port=21
  Outport_22 : Outport  Port=22
  Outport_23 : Outport  Port=23
  Outport_24 : Outport  Port=24
  Outport_25 : Outport  Port=25
  Outport_26 : Outport  Port=26
  Outport_27 : Outport  Port=27
  Outport_28 : Outport  Port=28
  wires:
  Inport_1/1 -> SigSpec_1/1
  SigSpec_1/1 -> Outport_1/1
  Inport_2/1 -> SigSpec_2/1
  SigSpec_2/1 -> Outport_2/1
  Inport_3/1 -> SigSpec_3/1
  SigSpec_3/1 -> Outport_3/1
  Inport_4/1 -> SigSpec_4/1
  SigSpec_4/1 -> Outport_4/1
  Inport_5/1 -> SigSpec_5/1
  SigSpec_5/1 -> Outport_5/1
  Inport_6/1 -> SigSpec_6/1
  SigSpec_6/1 -> Outport_6/1
  Inport_7/1 -> SigSpec_7/1
  SigSpec_7/1 -> Outport_7/1
  Inport_8/1 -> SigSpec_8/1
  SigSpec_8/1 -> Outport_8/1
  Inport_9/1 -> SigSpec_9/1
  SigSpec_9/1 -> Outport_9/1
  Inport_10/1 -> SigSpec_10/1
  SigSpec_10/1 -> Outport_10/1
  Inport_11/1 -> SigSpec_11/1
  SigSpec_11/1 -> Outport_11/1
  Inport_12/1 -> SigSpec_12/1
  SigSpec_12/1 -> Outport_12/1
  Inport_13/1 -> SigSpec_13/1
  SigSpec_13/1 -> Outport_13/1
  Inport_14/1 -> SigSpec_14/1
  SigSpec_14/1 -> Outport_14/1
  Inport_15/1 -> SigSpec_15/1
  SigSpec_15/1 -> Outport_15/1
  Inport_16/1 -> SigSpec_16/1
  SigSpec_16/1 -> Outport_16/1
  Inport_17/1 -> SigSpec_17/1
  SigSpec_17/1 -> Outport_17/1
  Inport_18/1 -> SigSpec_18/1
  SigSpec_18/1 -> Outport_18/1
  Inport_19/1 -> SigSpec_19/1
  SigSpec_19/1 -> Outport_19/1
  Inport_20/1 -> SigSpec_20/1
  SigSpec_20/1 -> Outport_20/1
  Inport_21/1 -> SigSpec_21/1
  SigSpec_21/1 -> Outport_21/1
  Inport_22/1 -> SigSpec_22/1
  SigSpec_22/1 -> Outport_22/1
  Inport_23/1 -> SigSpec_23/1
  SigSpec_23/1 -> Outport_23/1
  Inport_24/1 -> SigSpec_24/1
  SigSpec_24/1 -> Outport_24/1
  Inport_25/1 -> SigSpec_25/1
  SigSpec_25/1 -> Outport_25/1
  Inport_26/1 -> SigSpec_26/1
  SigSpec_26/1 -> Outport_26/1
  Inport_27/1 -> SigSpec_27/1
  SigSpec_27/1 -> Outport_27/1
  Inport_28/1 -> SigSpec_28/1
  SigSpec_28/1 -> Outport_28/1
